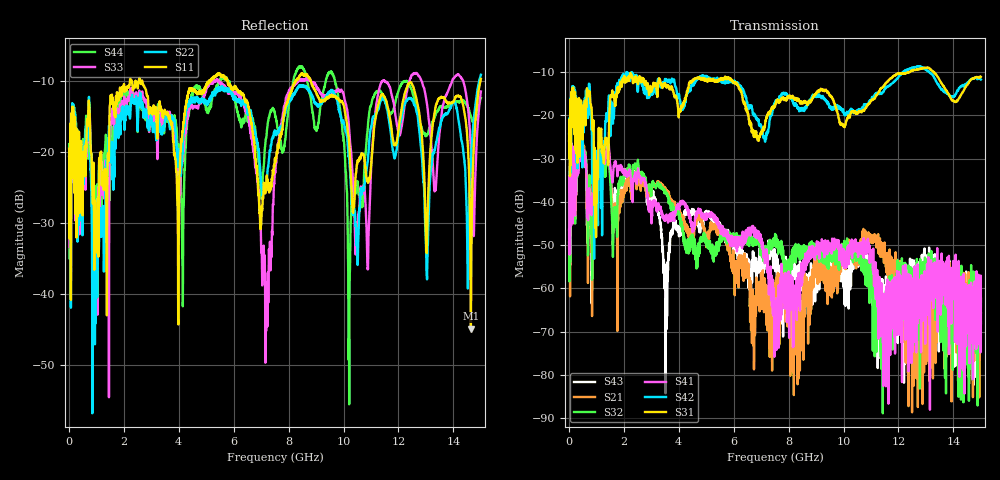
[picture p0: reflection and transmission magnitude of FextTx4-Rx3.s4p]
! FILE: N:\QM 2007\Prüfprotokolle\Highspeed\Konfektionierte Ltg\L45593-D106\D30\8216\0002\Fext\FextTx4-Rx3.s4p
# MHz S RI R 50.00
! FREQ  S11  S12  S13  S14
!  S21  S22  S23  S24
!  S31  S32  S33  S34
!  S41  S42  S43  S44
!  REAL  IMAG  REAL  IMAG  REAL  IMAG  REAL  IMAG
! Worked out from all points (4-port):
!   2999 points, 10 MHz to 15 GHz, reference 50 ohm
!   strongest paths, dB at 10 MHz, 3.755 GHz, 7.505 GHz, 11.26 GHz, 15 GHz:
!     S31: -25.8, -13.4, -18.0, -14.9, -11.1
!     S42: -24.4, -11.6, -17.3, -15.0, -11.8
!     S41: -46.4, -44.1, -63.0, -59.3, -68.1
!     S32: -40.9, -41.4, -47.8, -66.9, -64.1
!     S21: -50.5, -39.7, -66.7, -48.0, -65.8
!     S43: -49.4, -47.6, -53.8, -63.2, -62.4
!   lowest |S11| = -44.9 dB at 14.63 GHz (marker M1), VSWR 1.01, Z = 49.8 - j0.548 ohm
!   |S11| at or under -10 dB: 2.673 GHz to 5.107 GHz (2.434 GHz wide, 62.6 % of centre); 5.781 GHz to 8.261 GHz (2.48 GHz wide, 35.3 % of centre); 8.799 GHz to 14.98 GHz (6.182 GHz wide, 52 % of centre)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
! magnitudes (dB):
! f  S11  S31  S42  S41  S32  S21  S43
! 10 MHz  -19.5  -25.8  -24.4  -46.4  -40.9  -50.5  -49.4
! 455 MHz  -20.7  -19.9  -24.1  -30.7  -30.0  -29.4  -30.6
! 5.435 GHz  -9.1  -11.8  -11.7  -45.2  -49.3  -45.9  -44.9
! 7.205 GHz  -23.3  -20.6  -24.1  -52.6  -51.7  -62.5  -51.5
! 8.225 GHz  -10.2  -16.2  -17.3  -59.7  -50.4  -75.3  -54.4
! 14.63 GHz  -44.9  -11.8  -11.7  -68.7  -78.6  -70.6  -68.0
! 15 GHz  -9.7  -11.1  -11.8  -68.1  -64.1  -65.8  -62.4
